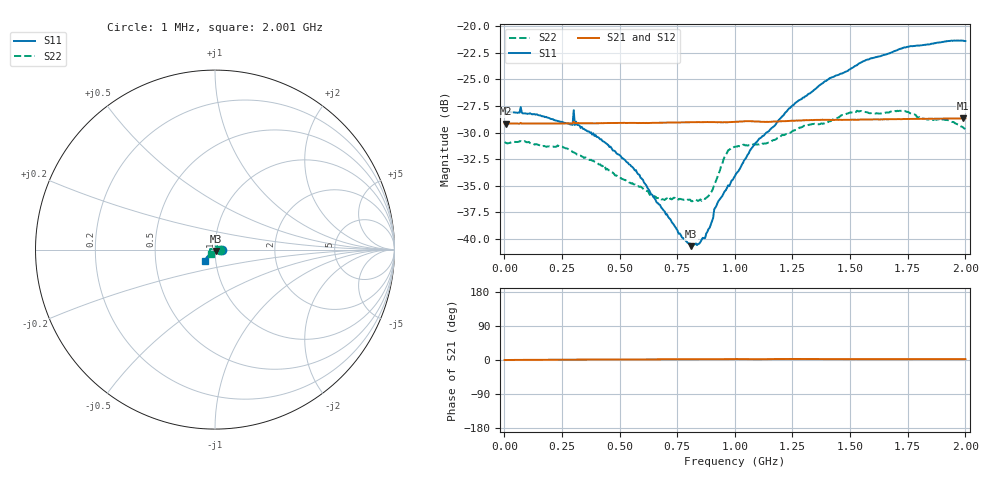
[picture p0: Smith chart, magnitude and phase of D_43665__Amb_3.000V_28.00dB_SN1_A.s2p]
! device id: 43665_
! dir: \\malibu\benchdata\1_engineers\tn_data\43665_75ohm\new\sparar\43665_\amb\3p000v\28p00db
! Serial: 1
! Insertion: A
! Temp: Amb
! VDD: 3.000V
! Attenuation Step: 28.00dB
! IDD: 1.449793e+00mA
! FILE NAME
! DATE 03-27-2009 08:40:16
! CORRECTED  DATA
#  Hz  S  RI  R  75
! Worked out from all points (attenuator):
!   401 points, 1 MHz to 2.001 GHz, reference 75 ohm
!   highest |S21| = -28.66 dB at 1.991 GHz (marker M1); lowest = -29.2 dB at 6 MHz (marker M2)
!   lowest |S11| = -40.7 dB at 811 MHz (marker M3), VSWR 1.02, Z = 75.6 - j1.25 ohm
!   |S11| at or under -10 dB: start of sweep to end of sweep
!   |S22| runs from -36.4 to -27.9 dB; largest |S21 - S12| = 0.00058
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1000000  0.0401 -0.000399  0.0349 3.64e-05  0.035 -3.2e-05  0.0285 -9.6e-05
6000000  0.04 -0.000576  0.0348 -8.35e-05  0.0347 2.57e-06  0.0283 -6.87e-06
2.41e8  0.0355 -0.000319  0.0349 0.000473  0.0349 0.000484  0.0247 0.0115
3.11e8  0.0356 -0.000715  0.0351 0.000612  0.0349 0.000609  0.0206 0.0145
3.36e8  0.0336 -0.000337  0.035 0.000612  0.035 0.000665  0.0195 0.0148
5.61e8  0.0213 -0.00258  0.0351 0.000866  0.0351 0.000928  0.00579 0.0171
6.71e8  0.0137 -0.00489  0.0352 0.00113  0.0352 0.00119  -0.0012 0.0155
7.66e8  0.00756 -0.00721  0.0353 0.00122  0.0353 0.0013  -0.00744 0.0135
8.11e8  0.00414 -0.00829  0.0353 0.00123  0.0353 0.00136  -0.0106 0.0108
8.46e8  0.00164 -0.00939  0.0354 0.00124  0.0354 0.00132  -0.0127 0.00847
8.91e8  -0.00221 -0.0111  0.0354 0.0012  0.0354 0.00135  -0.0155 0.00494
9.21e8  -0.00565 -0.0132  0.0354 0.00122  0.0354 0.00135  -0.0189 0.0028
9.61e8  -0.00844 -0.0147  0.0353 0.00137  0.0354 0.00149  -0.0247 0.00262
1.001e9  -0.0117 -0.016  0.0355 0.0015  0.0355 0.00163  -0.0268 0.00413
1.096e9  -0.0202 -0.0203  0.0356 0.00125  0.0357 0.00142  -0.0278 -0.000343
1.241e9  -0.0307 -0.0277  0.0358 0.00166  0.0359 0.00182  -0.0303 -0.00876
1.336e9  -0.0366 -0.0331  0.0362 0.00159  0.0363 0.00175  -0.032 -0.0133
1.526e9  -0.0477 -0.0445  0.0363 0.00146  0.0365 0.00162  -0.0326 -0.0224
1.671e9  -0.0527 -0.0526  0.0365 0.00146  0.0366 0.00159  -0.0302 -0.0252
1.916e9  -0.0565 -0.063  0.0368 0.00152  0.0369 0.00167  -0.0244 -0.0269
1.991e9  -0.0557 -0.0647  0.0369 0.00154  0.037 0.0016  -0.0212 -0.0259
2.001e9  -0.0555 -0.0644  0.0368 0.00157  0.0369 0.00159  -0.0209 -0.0254
